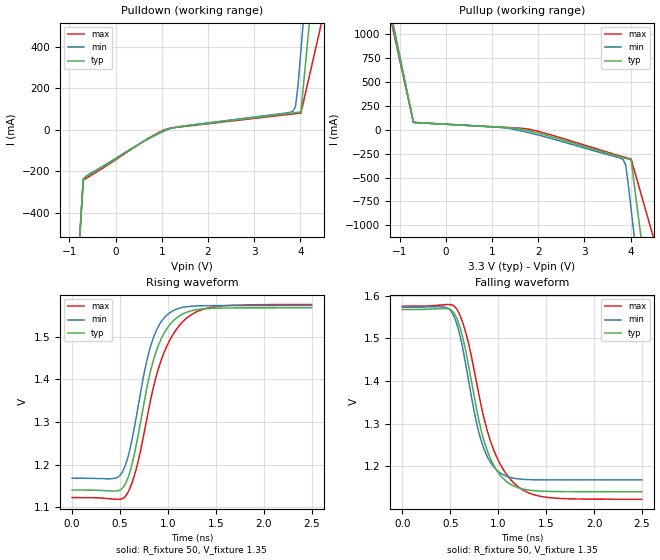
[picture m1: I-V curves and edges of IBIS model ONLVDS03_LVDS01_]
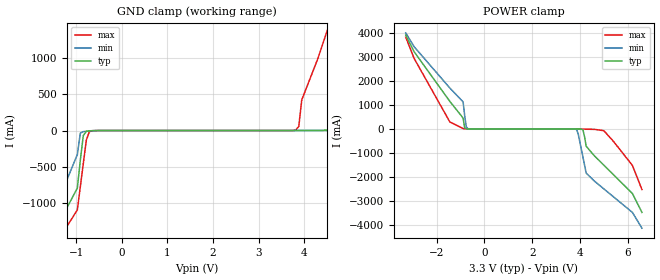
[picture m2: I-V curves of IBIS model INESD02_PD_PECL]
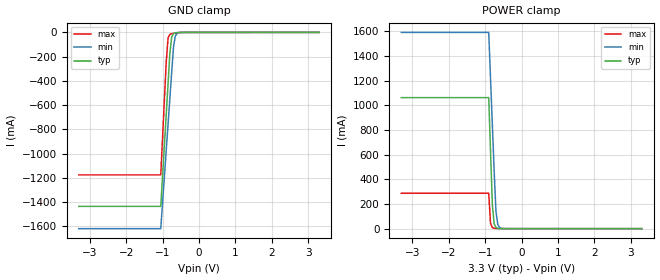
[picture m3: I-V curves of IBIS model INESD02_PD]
|   This file is an IBIS representation of the   |
|   Integrated Devices Technology, Inc.   |
|   ICS874003-05   |
|   PCI EXPRESS JITTER ATTENUATOR   |
[IBIS Ver]   4.1
[File name]   874003_05_3v3.ibs
[File Rev]   1.0
[Date]   9 Mar 2010
[Source]   Originated at Integrated Device Technology, Inc.
[Disclaimer]
IDT hereby grants the user of this IBIS model a non-exclusive,
nontransferable license to use this IBIS model under the following terms.
Before using this IBIS model, the user should read this license.
If the user does not accept these terms,  the IBIS model should be
returned to IDT within 30 days.
   The user is granted this license only to use the IBIS model and
is not granted rights to sell, load, rent, lease or license the IBIS
model in whole or in part, or in modified form to anyone other than
user. User may modify the IBIS model to suit its specific
applications but rights to derivative works and such modifications
shall belong to IDT.
   This IBIS model is provided on an "AS IS" basis and IDT makes
absolutely no warranty with respect to the information contained
herein. IDT DISCLAIMS AND CUSTOMER WAIVES ALL WARRANTIES, EXPRESS
OR IMPLIED, INCLUDING WARRANTIES OF MERCHANTABILITY OR FITNESS FOR
A PARTICULAR PURPOSE. The entire risk as to quality and performance
is with the Customer. ACCORDINGLY, IN NO EVENT SHALL THE COMPANY BE
LIABLE FOR ANY DAMAGES, WHETHER IN CONTRACT OR TORT,INCLUDING ANY
LOST PROFITS OR OTHER INCIDENTAL, CONSEQUENTIAL, EXEMPLARY, OR
PUNITIVE DAMAGES ARISING OUT OF THE USE OR APPLICATION OF THE IBIS
model provided in this package. Further, IDT reserves the right to
make changes without notice to any product herein to improve
reliability, function, or design. IDT does not convey any license
under patent rights or any other intellectual property rights,
including those of third parties.
   IDT is not obligated to provide maintenance or support
for the licensed IBIS model.
[Copyright]   Copyright 2010 by Integrated Device Technology , Inc.
[Component]   ICS874003G-05
[Manufacturer] Integrated Device Technology, Inc.
[Package]
|TSSOP 20 Lead
|   typ   min   max
R_pkg   51.85m   41.1m   62.6m
L_pkg   1.568nH   0.734nH   2.401nH
C_pkg   0.221pF   0.068pF   0.373pF
[Pin]   signal_name   model_name   R_pin   L_pin   C_pin
1   QA1   ONLVDS03_LVDS01_   62.6m   2.401n   0.373p
2   VDDO   POWER   57.23m   1.985n   0.297p
3   QA0   ONLVDS03_LVDS01_   51.85m   1.568n   0.221p
4   nQA0   ONLVDS03_LVDS01_   46.78m   1.151n   0.145p
5   MR   INESD02_PD_PECL   41.1m   0.734n   0.068p
6   FSEL_0   INESD02_PD   41.1m   0.734n   0.068p
7   NC   NC   46.78m   1.151n   0.145p
8   VDDA   POWER   51.85m   1.568n   0.221p
9   F_SEL1   INESD02_PD   57.23m   1.985n   0.297p
10   VDD   POWER   62.6m   2.401n   0.373p
11   OEA   INESD02_PU   62.6m   2.401n   0.373p
12   CLK   INESD02_PD_PECL   57.23m   1.985n   0.297p
13   nCLK   INESD02_PU_PECL   51.85m   1.568n   0.221p
14   GND   GND   46.78m   1.151n   0.145p
15   OEB   INESD02_PU   41.1m   0.734n   0.068p
16   F_SEL2   INESD02_PD   41.1m   0.734n   0.068p
17   nQB0   ONLVDS03_LVDS01_   46.78m   1.151n   0.145p
18   QB0   ONLVDS03_LVDS01_   51.85m   1.568n   0.221p
19   VDDO   POWER   57.23m   1.985n   0.297p
20   nQA1   ONLVDS03_LVDS01_   62.6m   2.401n   0.373p
[Diff Pin]  inv_pin  vdiff tdelay_typ tdelay_min  tdelay_max
|INPUT
12   13   0.15 0  0  0
|OUTPUT
1   20   NA   0  0  0
18   17   NA   0  0  0
3   4   NA   0  0  0
| Models and submodels in the file (5): ONLVDS03_LVDS01_ (Output), INESD02_PD_PECL (Input), INESD02_PD (Input), INESD02_PU (Input), INESD02_PU_PECL (Input)
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[Model]   ONLVDS03_LVDS01_
Model_type   Output
Polarity   Non-Inverting
|   typ   min   max
C_comp   2pF   1.5pF   2.5pF
Vmeas = 1.35V
Rref = 50
Cref = 0
Vref = 1.35V
|   typ   min   max
[Voltage range]   3.3V   3.135V   3.465V
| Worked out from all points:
|   slope of the pulldown table from 0 to 0.495 V, typ, clamps not added: 7.11 ohm
|   slope of the pullup table from 0 to 0.495 V, typ, clamps not added: 37.1 ohm
|   rising waveform, R_fixture 50, V_fixture 1.35: 20-80 % time 254ps typ, 223ps min, 308ps max; typ from 1.14 V to 1.57 V
|   falling waveform, R_fixture 50, V_fixture 1.35: 20-80 % time 254ps typ, 223ps min, 308ps max; typ from 1.57 V to 1.14 V
[Pulldown]
|Voltage   I (typ)   I (min)   I (max)
-3.3V     -12.71A    -11A       -15.57A
-1.22V    -2.155A    -2.204A    -2.106A
-700mV    -235.2mA   -238.7mA   -242.9mA
-591mV    -220.6mA   -216.2mA   -228mA
921.3mV   -16.78mA   -19.99mA   -14.52mA
1.353V    13.73mA    14.34mA    12.36mA
3.838V    80.83mA    89.88mA    76.17mA
3.892V    82.33mA    110.9mA    77.56mA
3.946V    83.9mA     210.5mA    78.94mA
4.01V     86.04mA    381.7mA    80.59mA
4.528V    1.295A     1.772A     585.3mA
6.6V      7.985A     7.362A     9.101A
[Pullup]
|Voltage   I (typ)   I (min)   I (max)
-3.3V     7.976A     6.908A     9.771A
-1.22V    1.261A     1.299A     1.219A
-700mV    77.19mA    81.44mA    75.57mA
1.191V    25.75mA    22.97mA    26.97mA
1.732V    -4.649mA   -23.29mA   10.34mA
3.784V    -285.3mA   -298.4mA   -275.7mA
3.838V    -292.4mA   -313.3mA   -283.2mA
3.892V    -299.5mA   -366mA     -290.6mA
3.946V    -306.6mA   -560.2mA   -297.9mA
4.01V     -315.3mA   -828.8mA   -306.6mA
4.528V    -2.273A    -3.003A    -1.186A
6.6V      -12.73A    -11.74A    -14.49A
[Ramp]
|   typ   min   max
dV/dt_r   0.343/0.406n   0.324/0.353n   0.364/0.497n
dV/dt_f   0.343/0.406n   0.324/0.353n   0.364/0.497n
R_load =   50.0000
[Rising Waveform]
R_fixture = 50
V_fixture = 1.35   |Vcc_typ
V_fixture_min = 1.365 |Vcc_min
V_fixture_max = 1.35 |Vcc_max
C_fixture = 0.0p
| Time   typ   min   max
0s        1.141V     1.169V     1.123V
455.5ps   1.139V     1.169V     1.119V
573.1ps   1.164V     1.211V     1.132V
678.2ps   1.257V     1.324V     1.199V
813.3ps   1.415V     1.474V     1.346V
908.4ps   1.484V     1.527V     1.431V
1.019ns   1.528V     1.556V     1.492V
1.184ns   1.556V     1.57V      1.541V
1.399ns   1.565V     1.572V     1.566V
2.498ns   1.567V     1.573V     1.575V
[Falling Waveform]
R_fixture = 50
V_fixture = 1.35   |Vcc_typ
V_fixture_min = 1.365 |Vcc_min
V_fixture_max = 1.35 |Vcc_max
C_fixture = 0.0p
| Time   typ   min   max
0s        1.567V     1.573V     1.575V
455.5ps   1.57V      1.572V     1.579V
573.1ps   1.544V     1.53V      1.567V
678.2ps   1.451V     1.418V     1.5V
813.3ps   1.293V     1.267V     1.352V
908.4ps   1.224V     1.214V     1.267V
1.019ns   1.18V      1.186V     1.207V
1.184ns   1.152V     1.172V     1.157V
1.399ns   1.143V     1.169V     1.132V
2.498ns   1.141V     1.168V     1.123V
[Model]   INESD02_PD_PECL
Model_type  Input
Polarity   Non-Inverting
Vinl = 0.8V
Vinh = 2.0V
|   typ   min   max
C_comp   2pF   1.5pF   2.5pF
|   typ   min   max
[Voltage range]  3.3V   3.15V   3.45V
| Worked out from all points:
|   GND clamp passes 1 mA (typ) near -0.59 V on its own axis
|   POWER clamp passes 1 mA (typ) near -0.70 V on its own axis
[GND_clamp]
-3.3V     -3.894A    -4.294A    -3.674A
-1.6V     -1.569A    -1.322A    -1.74A
-974.8mV  -794.1mA   -331.5mA   -1.096A
-843.4mV  -68.33mA   -15.34mA   -452.9mA
-646.5mV  -1.912mA   -4.151mA   -2.665mA
3.818V    89.38uA    70.49uA    7.198mA
3.95V     342.2uA    75.94uA    423.8mA
4.6V      7.437mA    165.5uA    1.553A
4.9V      78.32mA    440.9uA    2.118A
5.5V      1.293A     2.769mA    3.249A
6.25V     2.651A     112.4mA    4.38A
6.6V      3.331A     896.1mA    4.946A
[POWER_clamp]
-3.3V     3.923A     4.017A     3.838A
-2.95V    3.23A      3.44A      2.951A
-1.45V    1.149A     1.709A     289.6mA
-896.9mV  456.5mA    1.133A     15.4mA
-762.9mV  4.223mA    91.07mA    1.486mA
-695.9mV  792.2uA    10.73mA    555.6uA
3.861V    -556.7uA   -26.14mA   -39.45uA
4.129V    -41.85mA   -1.19A     -4.904mA
4.263V    -724.2mA   -1.847A    -12.04mA
5V        -1.514A    -2.505A    -71.38mA
6.2V      -2.701A    -3.492A    -1.525A
6.6V      -3.492A    -4.151A    -2.536A
[Model]   INESD02_PD
Model_type   Input
Polarity   Non-Inverting
Vinl = 0.80V
Vinh = 2.0V
|   typ   min   max
C_comp   2pF   1.5pF   2.5pF
|   typ   min   max
[Voltage range]  3.3V   3.15V   3.45V
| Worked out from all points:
|   GND clamp passes 1 mA (typ) near -0.56 V on its own axis
|   POWER clamp passes 1 mA (typ) near -0.61 V on its own axis
[GND_clamp]
|Voltage   I(typ)   I(min)   I(max)
-3.3V     -1.436A    -1.62A     -1.176A
-1.05V    -1.436A    -1.62A     -1.176A
-900mV    -678.5mA   -975.1mA   -244mA
-850mV    -426.1mA   -760.1mA   -46.85mA
-800mV    -173.9mA   -545.4mA   -16.11mA
-750mV    -36.96mA   -330.7mA   -9.916mA
-700mV    -9.696mA   -120.2mA   -7.056mA
-650mV    -3.545mA   -29.7mA    -4.857mA
-600mV    -1.629mA   -7.52mA    -3.049mA
-400mV    -52.81uA   -52.52uA   -108.7uA
3.3V      71.13uA    77.43uA    62.11uA
[POWER_clamp]
|Voltage   I(typ)   I(min)   I(max)
-3.3V     1.063A     1.593A     287.3mA
-900mV    1.063A     1.593A     287.3mA
-850mV    620.5mA    1.215A     41.84mA
-800mV    191.6mA    837.5mA    8.757mA
-750mV    37.76mA    460.2mA    3.328mA
-700mV    8.104mA    133.8mA    1.728mA
-650mV    2.076mA    32.66mA    905.3uA
-600mV    678.1uA    8.083mA    443.8uA
-450mV    104.2uA    213.3uA    89.09uA
3.3V      -3.041nA   -3.986uA   0A
